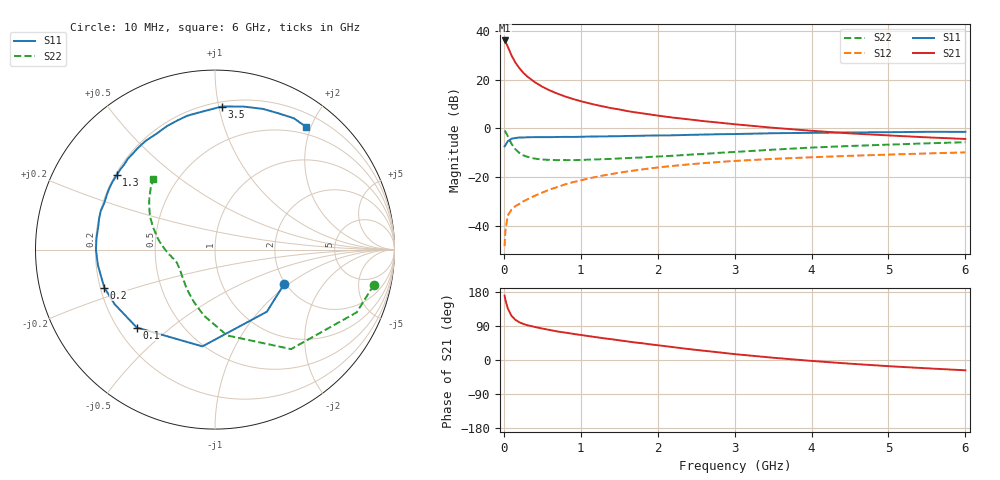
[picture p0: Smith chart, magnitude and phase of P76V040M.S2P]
! SIEMENS Small Signal Semiconductors
! BFP196
! Si NPN RF Bipolar Junction Transistor in SOT143
! VCE = 6 V  IC = 40 mA
! Common Emitter S-Parameters:  May  1996
# GHz  S  MA  R  50
!  f  S11  S21  S12  S22
! GHz  MAG  ANG  MAG  ANG  MAG  ANG  MAG  ANG
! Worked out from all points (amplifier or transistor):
!   36 points, 10 MHz to 6 GHz, reference 50 ohm
!   highest |S21| = 36.2 dB at 10 MHz (marker M1)
!   |S21| within 3 dB of that: start of sweep to 57.2 MHz
!   unconditionally stable (mu >= 1): 517.5 MHz to 4.345 GHz
!   at 250 MHz: K = 0.77, MSG = 26.5 dB, |S12| = -30.0 dB
!   at 1.4 GHz: K = 1.09, MAG = 11.7 dB, |S12| = -18.7 dB
!   at 6 GHz: K = 0.98, MSG = 2.8 dB, |S12| = -9.8 dB
!   S11 on the Smith chart (normalised r, x): 10 MHz: 1.97, -0.92; 100 MHz: 0.28, -0.39; 200 MHz: 0.22, -0.16; 1.3 GHz: 0.21, +0.32; 3.5 GHz: 0.23, +1.02; 6 GHz: 0.39, +1.93
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0.01  0.4306 -26.2  64.53 169.7  0.0038 80.1  0.9068 -12.5
0.02  0.4508 -50.1  61.15 159.1  0.0078 71.8  0.8633 -23.9
0.05  0.5437 -97.4  48.56 136.8  0.016 57.7  0.6979 -52.6
0.1  0.6153 -135.1  31.78 116.4  0.0216 49.1  0.4828 -82.0
0.15  0.6369 -151.6  22.72 106.0  0.0253 45.7  0.3731 -99.5
0.2  0.6521 -161.1  17.56 99.7  0.028 47.3  0.3158 -111.6
0.25  0.653 -168.1  14.13 95.4  0.0315 49.9  0.2817 -121.2
0.3  0.6582 -172.6  11.89 92.1  0.0345 52.2  0.2629 -127.8
0.4  0.6632 180.0  9.015 87.3  0.0412 55.6  0.2402 -138.2
0.5  0.6635 174.5  7.214 83.0  0.0481 57.6  0.2297 -145.2
0.6  0.6627 169.3  6.024 79.1  0.0558 58.9  0.2254 -150.0
0.7  0.6684 164.9  5.182 75.2  0.0627 59.5  0.2236 -153.9
0.9  0.6693 157.2  4.031 69.1  0.0787 59.2  0.2236 -159.3
1.1  0.681 149.9  3.318 63.1  0.0936 58.0  0.2284 -163.0
1.3  0.687 142.8  2.814 57.3  0.1087 56.1  0.2339 -166.4
1.7  0.7041 130.5  2.155 46.4  0.137 51.4  0.2496 -172.3
2.2  0.7231 116.8  1.671 34.0  0.1704 44.7  0.275 -179.1
2.8  0.7615 101.7  1.317 20.1  0.2047 36.3  0.3156 171.0
3.5  0.7981 87.3  1.033 6.0  0.2369 26.6  0.3664 160.2
4.5  0.8283 71.1  0.793 -9.7  0.274 14.9  0.4361 147.2
5.5  0.8534 59.0  0.657 -21.9  0.3066 4.3  0.4946 136.4
6  0.8516 53.4  0.609 -27.2  0.322 -1.4  0.5218 131.2
